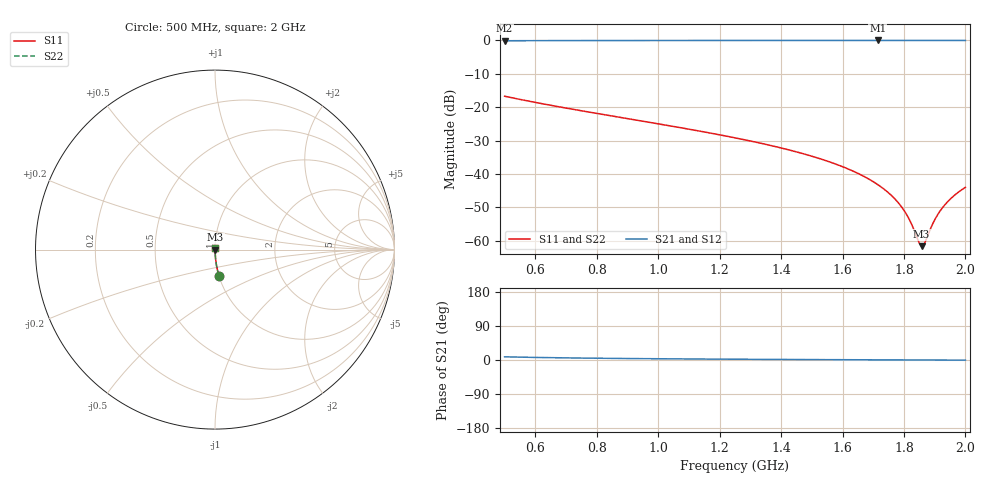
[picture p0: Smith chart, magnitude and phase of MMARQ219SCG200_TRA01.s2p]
! MMARQ219SCG200_TRA01  S-PARAMETER MODEL  ( General Type )
! Model Generated by TAIYO YUDEN Corporation (http://www.ty-top.com)
! Version 1.0
! TAIYO YUDEN Control No. 180601
! Copyright(c) 2018 TAIYO YUDEN CO.,LTD. All Rights Reserved.
! Product Description (link to TY-COMPAS)
! https://ds.yuden.co.jp/TYCOMPAS/or/detail?pn=MMARQ219SCG200JTRA01&u=M
! Products Name : Multilayer Ceramic Capacitors
! Characteristics :
!  Capacitance : 20 pF , Rated Voltage : 250V , TCC : CG / C0G
!  Case Size : 2.0 x 1.25 / 0.079 x 0.049 [mm/inch] , Thickness : 0.85 / 0.033 [mm/inch]
!  (Conditions: Temperature = 25 degC , DC Bias Current/Voltage = 0A / 0V)
! External Node Assignments :
!  1  o---| |---o  2
! GND o---------o GND
! Frequency Range : 500MHz  -  2000MHz  [ 401 STEP ]
# MHz S RI R 50
! Freq[MHz].  S11 Real  S11 Imag  S21 Real  S21 Imag  S12 Real  S12 Imag  S22 Real  S22 Imag
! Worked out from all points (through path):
!   401 points, 500 MHz to 2 GHz, reference 50 ohm
!   highest |S21| = -0.01 dB at 1.715 GHz (marker M1); lowest = -0.1 dB at 500 MHz (marker M2)
!   group delay of S21, straight-line fit = 14.1 ps
!   lowest |S11| = -61.6 dB at 1.857 GHz (marker M3), VSWR 1.00, Z = 50.1 - j0.00587 ohm
!   |S11| at or under -10 dB: start of sweep to end of sweep
!   |S22| runs from -61.6 to -16.7 dB; largest |S21 - S12| = 0
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500  0.0218 -0.1444  0.9782 0.1444  0.9782 0.1444  0.0218 -0.1444
751.25  0.00827 -0.0878  0.9917 0.0878  0.9917 0.0878  0.00827 -0.0878
1002.5  0.0037 -0.056  0.9963 0.056  0.9963 0.056  0.0037 -0.056
1250  0.00183 -0.0347  0.9982 0.0347  0.9982 0.0347  0.00183 -0.0347
1388.75  0.00131 -0.0252  0.9987 0.0252  0.9987 0.0252  0.00131 -0.0252
1501.25  0.00104 -0.0184  0.999 0.0184  0.999 0.0184  0.00104 -0.0184
1625  0.000879 -0.0115  0.9991 0.0115  0.9991 0.0115  0.000879 -0.0115
1673.75  0.000843 -0.00895  0.9992 0.00895  0.9992 0.00895  0.000843 -0.00895
1715  0.000824 -0.00687  0.9992 0.00687  0.9992 0.00687  0.000824 -0.00687
1752.5  0.000815 -0.00502  0.9992 0.00502  0.9992 0.00502  0.000815 -0.00502
1782.5  0.000813 -0.00357  0.9992 0.00357  0.9992 0.00357  0.000813 -0.00357
1805  0.000815 -0.0025  0.9992 0.0025  0.9992 0.0025  0.000815 -0.0025
1823.75  0.000818 -0.00162  0.9992 0.00162  0.9992 0.00162  0.000818 -0.00162
1850  0.000824 -0.000403  0.9992 0.000403  0.9992 0.000403  0.000824 -0.000403
1857.5  0.000827 -5.86e-05  0.9992 5.86e-05  0.9992 5.86e-05  0.000827 -5.86e-05
1861.25  0.000828 0.000113  0.9992 -0.000113  0.9992 -0.000113  0.000828 0.000113
1868.75  0.000831 0.000456  0.9992 -0.000456  0.9992 -0.000456  0.000831 0.000456
1898.75  0.000844 0.00181  0.9992 -0.00181  0.9992 -0.00181  0.000844 0.00181
1925  0.000859 0.00298  0.9991 -0.00298  0.9991 -0.00298  0.000859 0.00298
1958.75  0.000882 0.00446  0.9991 -0.00446  0.9991 -0.00446  0.000882 0.00446
1985  0.000903 0.0056  0.9991 -0.0056  0.9991 -0.0056  0.000903 0.0056
2000  0.000916 0.00624  0.9991 -0.00624  0.9991 -0.00624  0.000916 0.00624
